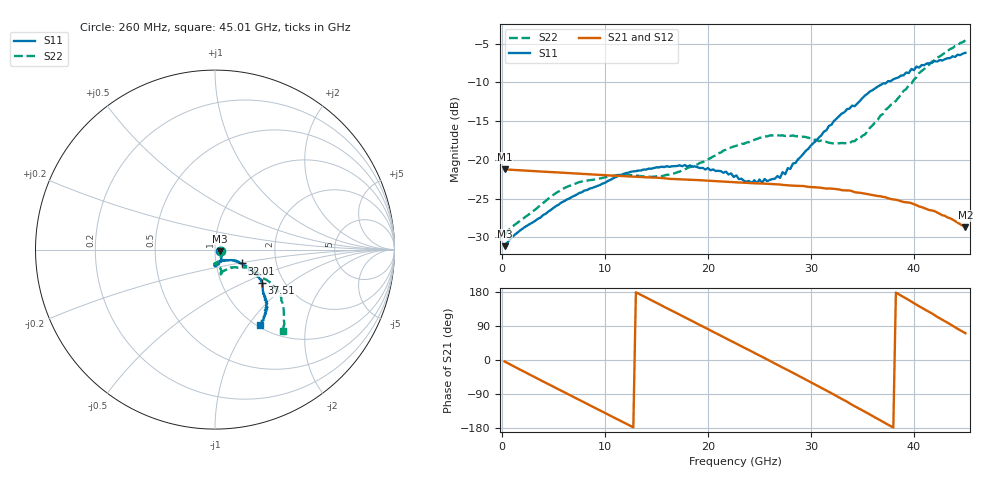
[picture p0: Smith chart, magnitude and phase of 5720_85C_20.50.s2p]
! Device:  ADRF5720
! Description: 0.5dB LSB GaAs MMIC 6-bit Digital Attenuator
! Frequency:  0.000009 -  40 GHz
! Ports:
!	RF1	= Port 1
!	RF2	= Port 2
! Vdd:  3.3 Volt
! Vss:  -3.3 Volt
! Control:  0/3.3 Volt
! State:  20.50 dB attenuation
! Data:  The device was measured using G-S-G Probes on a matrix board.
!  Data was collected using an calibrated 4 port network analyzer.
!  The reference plane for this measurement is at the launchers.
! Note:  Analog Devices supplies this data as a sample of measured data
!  for this product.  Your particular data for this product may vary.
!  Data was taken at 85 degrees C.
!  Analog Devices reserves the right to change this data at anytime.
# GHZ S DB R 45.0
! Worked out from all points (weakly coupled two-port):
!   180 points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, 260 MHz to 45.01 GHz, reference 45 ohm
!   highest |S21| = -21.23 dB at 260 MHz (marker M1); lowest = -28.7 dB at 45.01 GHz (marker M2)
!   lowest |S11| = -31.1 dB at 260 MHz (marker M3), VSWR 1.06, Z = 47.4 - j0.763 ohm
!   |S11| at or under -10 dB: start of sweep to 37.37 GHz
!   |S22| runs from -29.8 to -4.6 dB; largest |S21 - S12| = 0.00043
!   S11 on the Smith chart (normalised r, x): 260 MHz: 1.05, -0.02; 32.01 GHz: 1.33, -0.21; 37.51 GHz: 1.55, -0.64; 45.01 GHz: 1.03, -1.14
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0.26  -31.14 -16.8  -21.23 -3.9  -21.23 -3.9  -29.75 -15.6
1.76  -29.11 -6.7  -21.35 -25.4  -21.34 -25.3  -27.87 -19.1
5.26  -25.96 -41.7  -21.61 -74.1  -21.60 -74.1  -24.27 -65.1
7.76  -24.18 -55.7  -21.80 -108.7  -21.79 -108.6  -22.80 -80.3
12.01  -21.71 -74.8  -22.11 -167.4  -22.10 -167.2  -21.91 -92.6
15.26  -20.97 -85.2  -22.33 147.3  -22.32 147.5  -22.11 -88.7
18.26  -20.72 -90.3  -22.57 105.9  -22.56 106.0  -20.94 -79.2
22.76  -22.01 -84.0  -22.90 43.2  -22.88 43.5  -18.18 -73.8
24.26  -23.00 -76.1  -23.02 22.5  -23.00 22.7  -17.55 -74.9
27.01  -22.32 -50.4  -23.18 -16.3  -23.17 -16.0  -16.86 -76.5
27.26  -21.59 -46.7  -23.23 -19.9  -23.21 -19.7  -16.84 -77.3
27.51  -21.85 -45.9  -23.26 -23.3  -23.25 -23.1  -16.92 -76.9
27.76  -21.07 -42.2  -23.28 -26.8  -23.27 -26.6  -16.82 -77.8
28.01  -21.16 -42.4  -23.31 -30.4  -23.30 -30.1  -16.91 -77.5
30.26  -17.83 -30.2  -23.52 -62.5  -23.51 -62.2  -17.43 -76.3
32.01  -15.45 -27.3  -23.71 -87.8  -23.70 -87.5  -17.84 -68.7
34.76  -12.40 -30.4  -24.24 -129.1  -24.22 -128.8  -17.27 -46.3
37.51  -9.84 -35.4  -24.96 -171.1  -24.94 -170.7  -13.28 -28.1
37.76  -9.84 -35.8  -25.05 -174.7  -25.04 -174.4  -12.91 -28.3
41.51  -7.53 -47.2  -26.48 126.7  -26.46 127.0  -7.69 -32.8
43.51  -6.87 -51.4  -27.54 94.8  -27.51 95.1  -5.70 -42.3
45.01  -6.18 -59.3  -28.70 70.7  -28.66 71.1  -4.59 -50.0
